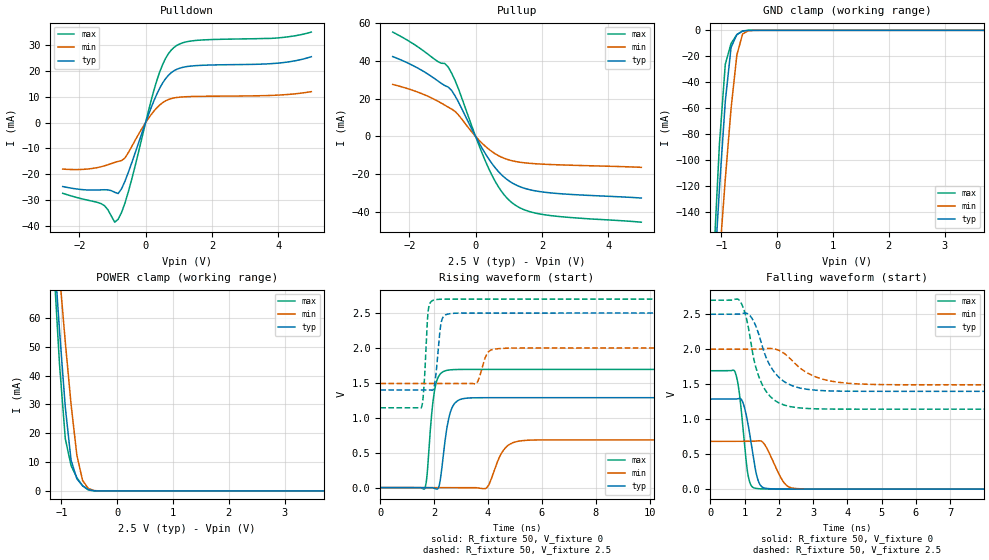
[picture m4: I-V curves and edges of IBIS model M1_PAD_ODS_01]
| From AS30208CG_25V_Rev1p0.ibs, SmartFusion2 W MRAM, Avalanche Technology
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[Model] M1_PAD_ODS_01
Model_type I/O
Enable   Active-High
Vinl  =  0.7
Vinh  =  1.8
Vmeas =  1.25
Cref  =  30e-12
| Capacitance   typ   min   max
C_comp   1.569373e-12  1.477665e-12  1.713725e-12
| Variables   typ   min   max
[GND Clamp Reference]   0   0   0
[POWER Clamp Reference]   2.5   2   2.7
[Pulldown Reference]   0   0   0
[Pullup Reference]   2.5   2   2.7
[Temperature Range]   25   125   -40
[Voltage Range]   2.5   2   2.7
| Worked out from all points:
|   slope of the pulldown table from 0 to 0.375 V, typ, clamps not added: 31.1 ohm
|   slope of the pullup table from 0 to 0.375 V, typ, clamps not added: 33 ohm
|   GND clamp passes 1 mA (typ) near -0.64 V on its own axis
|   POWER clamp passes 1 mA (typ) near -0.56 V on its own axis
|   falling waveform, R_fixture 50, V_fixture 0: 20-80 % time 264ps typ, 402ps min, 209ps max; typ from 1.29 V to 0 V
|   falling waveform, R_fixture 50, V_fixture 2.5: 20-80 % time 593ps typ, 887ps min, 479ps max; typ from 2.5 V to 1.4 V
|   rising waveform, R_fixture 50, V_fixture 0: 20-80 % time 286ps typ, 464ps min, 230ps max; typ from 0 V to 1.29 V
|   rising waveform, R_fixture 50, V_fixture 2.5: 20-80 % time 162ps typ, 249ps min, 125ps max; typ from 1.4 V to 2.5 V
[GND Clamp]
| Voltage   I(typ)   I(min)   I(max)
-2.5V     -1.297A    -1.146A    -1.538A
-1.138V   -196mA     -238.3mA   -175.4mA
-1.034V   -121.2mA   -175.1mA   -86.76mA
-931mV    -54.83mA   -114.9mA   -26.21mA
-827.6mV  -13.18mA   -60.42mA   -10.12mA
-724.1mV  -3.226mA   -19.15mA   -3.372mA
-620.7mV  -623.1uA   -2.801mA   -433.9uA
-517.2mV  -35.15uA   -320.3uA   -7.309uA
-413.8mV  -841.1nA   -24.53uA   -57.63nA
5V        0A         0A         0A
[POWER Clamp]
| Voltage   I(typ)   I(min)   I(max)
-2.5V     511mA      454.9mA    606.6mA
-1.138V   84.76mA    99.9mA     78.64mA
-1.034V   55.67mA    75.27mA    43.94mA
-931mV    29.07mA    51.7mA     18.16mA
-827.6mV  10.68mA    30.08mA    8.788mA
-724.1mV  4.238mA    12.45mA    4.618mA
-620.7mV  1.771mA    3.587mA    1.776mA
-517.2mV  465uA      837.9uA    329.7uA
-413.8mV  47.65uA    120.2uA    11.19uA
-310.3mV  1.515uA    11.72uA    116.8nA
5V        0A         0A         0A
[Pulldown]
| Voltage   I(typ)   I(min)   I(max)
-2.5V     -24.84mA   -18.06mA   -27.47mA
-1.345V   -26.13mA   -17.16mA   -31.47mA
-1.138V   -26.14mA   -16.38mA   -33.83mA
-931mV    -27.08mA   -15.46mA   -38.7mA
-827.6mV  -27.55mA   -15.06mA   -37.59mA
-517.2mV  -19.21mA   -11.59mA   -26.74mA
344.8mV   11.25mA    5.851mA    16.61mA
603.4mV   17.11mA    8.493mA    24.99mA
948.3mV   20.78mA    9.791mA    30.07mA
1.638V    22.25mA    10.22mA    32.08mA
3.99V     23.14mA    10.7mA     32.95mA
5V        25.64mA    12.06mA    35.21mA
[Pullup]
| Voltage   I(typ)   I(min)   I(max)
-2.5V     42.42mA    27.62mA    55.43mA
-1.552V   34.36mA    22.2mA     45.21mA
-827.6mV  26.25mA    15.56mA    36.93mA
-724.1mV  24.46mA    14.55mA    33.66mA
-517.2mV  18.3mA     11.42mA    25.3mA
86.21mV   -2.826mA   -1.658mA   -4mA
431mV     -12.85mA   -7.255mA   -18.38mA
775.9mV   -20.27mA   -10.97mA   -29.06mA
1.121V    -24.9mA    -13.01mA   -35.54mA
1.552V    -27.96mA   -14.16mA   -39.52mA
2.069V    -29.63mA   -14.78mA   -41.6mA
5V        -32.74mA   -16.44mA   -45.58mA
[Ramp]
dV/dt_r   0.772527/0.286359n  0.409943/0.464152n  1.01555/0.229639n
dV/dt_f   0.661206/0.592755n  0.305569/0.886872n  0.934102/0.478905n
R_load = 50
[Falling Waveform]
R_fixture = 50
V_fixture = 0
V_fixture_min = 0
V_fixture_max = 0
| Time   V(typ)   V(min)   V(max)
0s        1.288V     683.2mV    1.693V
734.4ps   1.288V     683.5mV    1.66V
865.6ps   1.296V     683.6mV    1.305V
1.093ns   954mV      683.6mV    228.9mV
1.194ns   653.1mV    683.7mV    51.59mV
1.332ns   244.9mV    687.1mV    11.43mV
1.549ns   21.43mV    662mV      3.007mV
2.165ns   1.126mV    84.99mV    476.1uV
2.557ns   755.1uV    6.767mV    466.6uV
21.88ns   2.004nV    168nV      -274.5nV
[Falling Waveform]
R_fixture = 50
V_fixture = 2.5
V_fixture_min = 2
V_fixture_max = 2.7
| Time   V(typ)   V(min)   V(max)
0s        2.5V       2V         2.7V
860.4ps   2.504V     2V         2.694V
1.062ns   2.513V     2.001V     2.428V
1.236ns   2.426V     2.001V     1.947V
1.563ns   1.968V     2.008V     1.45V
1.967ns   1.616V     1.991V     1.243V
2.538ns   1.455V     1.765V     1.164V
3.362ns   1.406V     1.561V     1.146V
4.729ns   1.398V     1.497V     1.144V
21.88ns   1.398V     1.491V     1.143V
[Rising Waveform]
R_fixture = 50
V_fixture = 0
V_fixture_min = 0
V_fixture_max = 0
| Time   V(typ)   V(min)   V(max)
0s        2.822nV    63.43nV    12.25nV
1.644ns   -240.3uV   -236.7uV   -18.25mV
2.027ns   -13.46mV   -291.9uV   1.418V
2.216ns   81.11mV    -319.2uV   1.621V
2.459ns   820.4mV    -354.2uV   1.679V
2.963ns   1.262V     -426.9uV   1.692V
3.943ns   1.287V     -4.109mV   1.693V
4.575ns   1.288V     537.1mV    1.693V
5.281ns   1.288V     672.9mV    1.693V
21.88ns   1.288V     683.2mV    1.693V
[Rising Waveform]
R_fixture = 50
V_fixture = 2.5
V_fixture_min = 2
V_fixture_max = 2.7
| Time   V(typ)   V(min)   V(max)
0s        1.398V     1.491V     1.143V
1.527ns   1.399V     1.491V     1.148V
1.621ns   1.399V     1.491V     1.441V
1.782ns   1.4V       1.491V     2.54V
2.055ns   1.585V     1.491V     2.692V
2.272ns   2.382V     1.491V     2.698V
2.6ns     2.492V     1.492V     2.699V
3.555ns   2.499V     1.489V     2.699V
4.487ns   2.499V     1.992V     2.699V
21.88ns   2.5V       2V         2.7V
